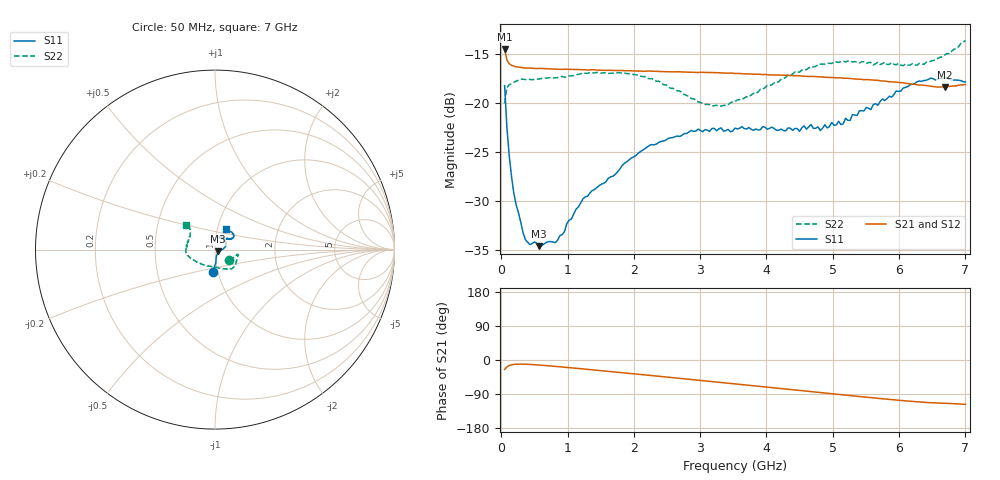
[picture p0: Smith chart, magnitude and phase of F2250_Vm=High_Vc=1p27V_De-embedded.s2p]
! Integrated Device Technology
! Corporate Headquarters
! 6024 Silver Creek Valley Road
! San Jose, CA 95138  USA
! Phone:  1-408-284-8200
! Toll Free:  1-800-223-1366
! Webpage:  http://www.idt.com/
! Timing and RF Division
! 515 Groton Road, Suite 102
! Westford, MA 01886-6024
! Device:  F2250
! Description: Voltage Variable RF Attenuator
! Frequency:  50.0 -  6000.00 MHz
! Package:  3x3 mm Thin QFN Plastic Package: 16 pin
! Ports:  2 RF, 3 DC
!  Pin  1  = GND
!  Pin  2  = NC
!  Pin  3  = RF1  = Port 1
!  Pin  4  = NC
!  Pin  5  = GND
!  Pin  6  = GND
!  Pin  7  = GND
!  Pin  8  = GND
!  Pin  9  = NC
!  Pin 10  = RF2  = Port 2
!  Pin 11  = NC
!  Pin 12  = GND
!  Pin 13  = GND
!  Pin 14  = VCNTRL
!  Pin 15  = VDD
!  Pin 16  = VMODE
! Vcntrl:  1.270 Volts
! Vmode:  +3.300 Volts
! Vdd:  +3.30  Volts
! Current:  1.332 mA
! Data:  The device was measured on a the F2250 evaluation board which has
!  individual transmission lines to the RF pins.  Data was collected
!  using a calibrated network analyzer.  The evaluation board was
!  de-embedded using a TRL calibration technique.
!  The reference plane is the edge of the package pin.
! Misc:  SN 10
!  Action Tracker AT0258
! Date Measured:  2014-11-26
! Date:  2015-10-15  MJV
! Note:
!  Integrated Device Technology supplies this data as a sample of measured
!  data at the package pin for this product.  Your particular data for this
!  product may vary.
!  Data was taken at 25 degrees C.
!  Integrated Device Technology reserves the right to change this data at anytime.
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# GHz S dB R 50
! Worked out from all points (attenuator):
!   201 points, 50 MHz to 7 GHz, reference 50 ohm
!   highest |S21| = -14.46 dB at 50 MHz (marker M1); lowest = -18.4 dB at 6.687 GHz (marker M2)
!   lowest |S11| = -34.6 dB at 571.2 MHz (marker M3), VSWR 1.04, Z = 51.7 - j0.913 ohm
!   |S11| at or under -10 dB: start of sweep to end of sweep
!   |S22| runs from -20.3 to -13.6 dB; largest |S21 - S12| = 0.00068
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0.05  -18.20 -95.9  -14.46 -25.0  -14.46 -25.0  -20.01 -37.0
0.08475  -22.48 -86.9  -15.59 -18.0  -15.58 -18.0  -18.42 -18.3
0.1195  -25.34 -83.6  -15.97 -14.5  -15.94 -14.5  -18.11 -13.3
0.189  -29.20 -75.0  -16.22 -11.6  -16.21 -11.6  -17.85 -11.8
0.22375  -30.38 -69.6  -16.28 -11.1  -16.26 -11.1  -17.76 -12.2
0.36275  -33.94 -51.6  -16.40 -11.1  -16.40 -11.1  -17.59 -13.3
0.57125  -34.60 -28.3  -16.45 -13.3  -16.45 -13.3  -17.54 -18.9
0.84925  -33.99 -18.7  -16.52 -17.4  -16.52 -17.4  -17.38 -26.9
1.2315  -29.75 -9.7  -16.59 -23.5  -16.56 -23.6  -16.93 -36.1
1.96125  -25.59 10.4  -16.69 -35.8  -16.70 -35.8  -17.01 -49.3
2.37825  -23.99 21.3  -16.77 -42.9  -16.77 -43.0  -17.75 -58.1
3.07325  -22.70 43.3  -16.86 -55.1  -16.86 -55.2  -20.13 -88.0
3.525  -22.55 57.7  -16.96 -63.1  -16.94 -63.2  -19.82 -118.8
4.7065  -22.57 65.7  -17.27 -84.0  -17.27 -84.1  -16.30 -166.3
5.15825  -22.09 48.4  -17.45 -92.0  -17.42 -92.1  -15.72 -175.6
5.193  -21.53 48.7  -17.44 -92.6  -17.44 -92.7  -15.78 -176.5
5.2625  -21.75 45.2  -17.48 -93.8  -17.47 -93.9  -15.69 -177.5
5.29725  -21.16 44.5  -17.50 -94.5  -17.49 -94.5  -15.79 -178.4
5.85325  -19.29 34.2  -17.81 -103.9  -17.80 -104.1  -16.03 167.6
6.3745  -17.68 36.9  -18.17 -111.7  -18.18 -111.8  -16.02 150.4
6.68725  -17.41 45.2  -18.36 -114.2  -18.37 -114.2  -15.08 141.1
7  -17.83 62.7  -18.09 -117.1  -18.09 -117.2  -13.59 139.7
